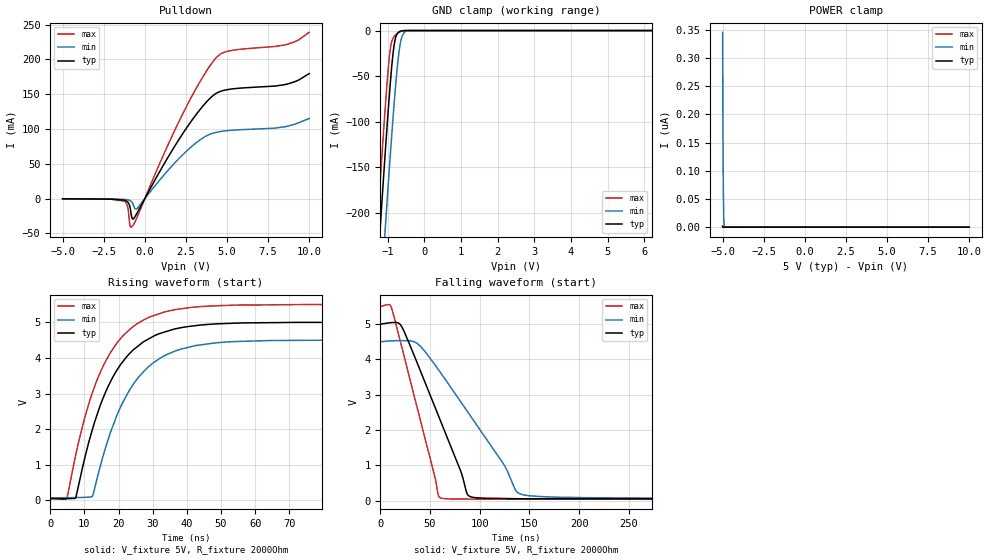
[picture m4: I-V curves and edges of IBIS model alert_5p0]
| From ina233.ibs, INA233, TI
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|   alert_5p0
[Model]   alert_5p0
Model_type   Open_drain
Polarity   Non-Inverting
Vmeas = 2.5
Vref = 5
Cref = 2pF
Rref = 2000
|   typ   min   max
C_comp   1.357E-12   1.334E-12   1.374E-12
| C_comp_pull_down   1.172E-12   1.078E-12   1.239E-12
| Where Nom  PVT is Nominal Process, 5V, 25C
|   Fast PVT is Strong Process,  5.5V, -40C
|   Slow PVT is Weak Process,   4.5V, 125C
[Voltage Range]   5   4.5   5.5
[Temperature Range]   25   125   -40
[Pullup Reference]   5   4.5   5.5
[Pulldown Reference]   -0   -0   -0
[Power Clamp Reference]   5   4.5   5.5
[GND Clamp Reference]   0   0   0
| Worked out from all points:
|   slope of the pulldown table from 0 to 0.75 V, typ, clamps not added: 23.2 ohm
|   GND clamp passes 1 mA (typ) near -0.67 V on its own axis
|   falling waveform, V_fixture 5V, R_fixture 2000Ohm: 20-80 % time 42.6ns typ, 65.1ns min, 29.7ns max; typ from 5 V to 0.054 V
|   rising waveform, V_fixture 5V, R_fixture 2000Ohm: 20-80 % time 12.5ns typ, 12.7ns min, 12.3ns max; typ from 0.054 V to 5 V
[Pulldown]
|   Voltage   I(typ)   I(min)   I(max)
-5V       -181.9uA   -109.6uA   -217.3uA
-1.25V    -2.203mA   -998.6uA   -3.554mA
-1.04V    -4.701mA   -1.635mA   -11.91mA
-920mV    -10.31mA   -2.468mA   -35.86mA
-815mV    -24.15mA   -4.099mA   -40.58mA
-710mV    -29.24mA   -8.24mA    -37.96mA
-485mV    -21.28mA   -14.42mA   -27.51mA
2.11V     86.16mA    58.4mA     112.3mA
4.3V      150.6mA    95.02mA    201.3mA
5.215V    157.2mA    98.06mA    212.6mA
8.695V    164.7mA    104.1mA    221.8mA
10V       179.5mA    115mA      238.8mA
[GND Clamp]
|   Voltage   I(typ)   I(min)   I(max)
-5V       -2.705A    -2.782A    -2.659A
-1.43V    -359.8mA   -444.6mA   -308.9mA
-1.25V    -246.6mA   -331.5mA   -195.5mA
-1.13V    -173mA     -257.4mA   -122.5mA
-1.085V   -146.1mA   -230.1mA   -96.18mA
-1.04V    -119.7mA   -203.1mA   -71.04mA
-935mV    -62.22mA   -141.7mA   -22.99mA
-800mV    -11.03mA   -69.29mA   -5.663mA
-650mV    -713.5uA   -13.46mA   -1.106mA
-545mV    -78.09uA   -2.061mA   -130.7uA
-410mV    -2.014uA   -80.45uA   -2.423uA
10V       0A         0A         0A
[POWER Clamp]
|   Voltage   I(typ)   I(min)   I(max)
-5V       758.9pA    345.5nA    2.565nA
-4.985V   379.4pA    194.2nA    1.282nA
-4.97V    0A         115.5nA    0A
-4.955V   0A         64.65nA    0A
-4.94V    0A         31.79nA    0A
-4.925V   0A         10.56nA    0A
-4.895V   0A         0A         0A
10V       0A         0A         0A
[Ramp]
R_load = 2000
|   typ   min   max
dV/dt_r   2.96781/1.24374e-08   2.6567/1.26566e-08   3.27309/1.23083e-08
dV/dt_f   2.96781/4.25718e-08   2.6567/6.50222e-08   3.27309/2.97108e-08
[Falling Waveform]
V_fixture = 5V
V_fixture_min = 4.5V
V_fixture_max = 5.5V
R_fixture = 2000Ohm
C_fixture = 0F
|   Time   V(typ)   V(min)   V(max)
0s        5V         4.5V       5.5V
11.52ns   5.029V     4.514V     5.425V
22.55ns   4.864V     4.52V      4.237V
37.98ns   3.832V     4.423V     2.532V
58.25ns   2.42V      3.709V     170.9mV
60.52ns   2.261V     3.62V      85.19mV
88.53ns   152.1mV    2.485V     51.3mV
136.4ns   62.92mV    290.8mV    47.57mV
142.4ns   61.44mV    181.4mV    47.52mV
500ns     53.65mV    72.16mV    44.85mV
[Rising Waveform]
V_fixture = 5V
V_fixture_min = 4.5V
V_fixture_max = 5.5V
R_fixture = 2000Ohm
C_fixture = 0F
|   Time   V(typ)   V(min)   V(max)
0s        53.65mV    72.16mV    44.85mV
4.849ns   54.44mV    78.38mV    45.67mV
7.451ns   73.56mV    81.72mV    1.275V
12.35ns   1.995V     120.4mV    3.032V
19.29ns   3.623V     2.335V     4.39V
23.13ns   4.115V     3.087V     4.789V
27.98ns   4.49V      3.683V     5.099V
40.94ns   4.888V     4.31V      5.415V
82.84ns   4.998V     4.499V     5.498V
500ns     5V         4.5V       5.5V
